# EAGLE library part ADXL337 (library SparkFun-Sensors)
Analog Devices ADXL337 3-Axis Analog Accelerometer The ADXL337 is a small, thin, low power, complete 3-axis accelerometer with signal conditioned voltage outputs. The product measures acceleration with a minimum full-scale range of ±3g. It can measure the static acceleration of gravity in tiltsensing applications, as well as dynamic acceleration resulting from motion, shock, or vibration. Datasheet SparkFun Products SparkFun Triple Axis Accelerometer Breakout - ADXL337 (SEN-12786)
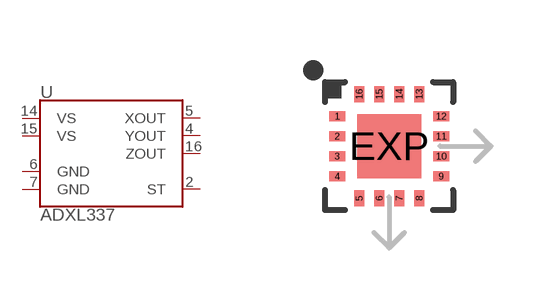
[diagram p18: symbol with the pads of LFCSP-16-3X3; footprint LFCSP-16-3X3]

Designator prefix U

## ADXL337 (PROD_ID: IC-12011)  [LFCSP-16-3X3]
2  ST
4  YOUT
5  XOUT
6  GND
7  GND
14  VS
15  VS
16  ZOUT

## Footprint LFCSP-16-3X3 (pad centres in mm)
16-Pin Lead Frame Chip Scale (LFCSP) w/ Center Pad (3 x 3 mm) Datasheet Specifications: Pin Count: 16 (+ center pad) Area: 3.0 x 3.0 x 1.45 mm Pitch: 0.5 mm Devices Using: ADXL337 ADXL377
smd 0.4 x 0.25: 1 -1.3,0.75; 2 -1.3,0.25; 3 -1.3,-0.25; 4 -1.3,-0.75; 9 1.3,-0.75; 10 1.3,-0.25; 11 1.3,0.25; 12 1.3,0.75
smd 0.25 x 0.4: 5 -0.75,-1.3; 6 -0.25,-1.3; 7 0.25,-1.3; 8 0.75,-1.3; 13 0.75,1.3; 14 0.25,1.3; 15 -0.25,1.3; 16 -0.75,1.3
smd 1.6 x 1.6: EXP 0,0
